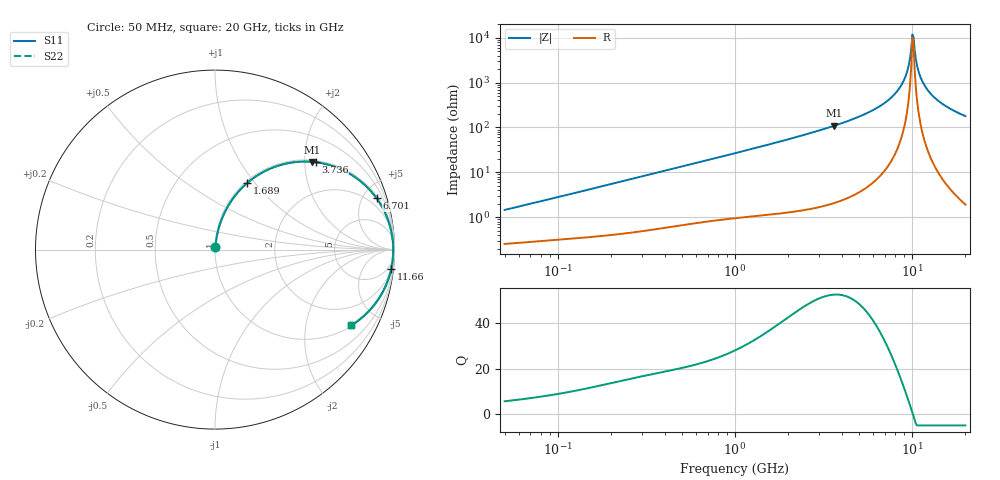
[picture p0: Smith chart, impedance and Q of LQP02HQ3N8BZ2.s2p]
!Murata Part Number: LQP02HQ3N8BZ2
!These Parameters are Measured in Series Mode Connection
!  o--[Z]--o
!Port1  Port2
!  o-------o
!Freq. Start=50[MHz] Stop=20[GHz], 401[Steps]
# Hz S RI R 50
!Freq.(Hz) S11(Real) S11(Imag) S21(Real) S21(Imag) S12(Real) S12(Imag) S22(Real) S22(Imag)
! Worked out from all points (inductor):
!   401 points, 50 MHz to 20 GHz, reference 50 ohm
!   read as one part in series: L = 4.53 nH near 51.52 MHz
!   highest Q = 52.5 at 3.626 GHz (marker M1), where L = 4.78 nH
!   self-resonance near 10.04 GHz
!   S11 on the Smith chart (normalised r, x): 50 MHz: 1.01, +0.03; 1.689 GHz: 1.02, +0.91; 3.736 GHz: 1.04, +2.26; 6.701 GHz: 1.18, +6.25; 11.66 GHz: 2, -18; 20 GHz: 1.04, -3.58
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5e7  0.00275 0.0143  0.9972 -0.0143  0.9972 -0.0143  0.00275 0.0143
1.364002e8  0.0049 0.0375  0.9951 -0.0375  0.9951 -0.0375  0.0049 0.0375
3.721004e8  0.0155 0.0989  0.9845 -0.0989  0.9845 -0.0989  0.0155 0.0989
1e9  0.0743 0.245  0.9257 -0.245  0.9257 -0.245  0.0743 0.245
1.689197e9  0.1787 0.3704  0.8213 -0.3704  0.8213 -0.3704  0.1787 0.3704
2.728004e9  0.3749 0.4741  0.6251 -0.4741  0.6251 -0.4741  0.3749 0.4741
3.626126e9  0.5416 0.4888  0.4584 -0.4888  0.4584 -0.4888  0.5416 0.4888
3.736399e9  0.5605 0.4869  0.4395 -0.4869  0.4395 -0.4869  0.5605 0.4869
5.194772e9  0.7683 0.4115  0.2317 -0.4115  0.2317 -0.4115  0.7683 0.4115
6.701223e9  0.9006 0.2853  0.0994 -0.2853  0.0994 -0.2853  0.9006 0.2853
7.442007e9  0.9405 0.2193  0.0595 -0.2193  0.0595 -0.2193  0.9405 0.2193
8.389408e9  0.973 0.1367  0.027 -0.1367  0.027 -0.1367  0.973 0.1367
9.041845e9  0.9856 0.0824  0.0144 -0.0824  0.0144 -0.0824  0.9856 0.0824
9.457416e9  0.9902 0.0492  0.00975 -0.0492  0.00975 -0.0492  0.9902 0.0492
9.892087e9  0.9926 0.0157  0.00741 -0.0157  0.00741 -0.0157  0.9926 0.0157
1.004137e10  0.9929 0.0045  0.00713 -0.0045  0.00713 -0.0045  0.9929 0.0045
1.034674e10  0.9927 -0.0179  0.00734 0.0179  0.00734 0.0179  0.9927 -0.0179
1.066139e10  0.9914 -0.0402  0.00857 0.0402  0.00857 0.0402  0.9914 -0.0402
1.098561e10  0.9892 -0.0625  0.0108 0.0625  0.0108 0.0625  0.9892 -0.0625
1.166392e10  0.9817 -0.1066  0.0183 0.1066  0.0183 0.1066  0.9817 -0.1066
1.438523e10  0.9254 -0.2515  0.0746 0.2515  0.0746 0.2515  0.9254 -0.2515
2e10  0.7597 -0.422  0.2403 0.422  0.2403 0.422  0.7597 -0.422
